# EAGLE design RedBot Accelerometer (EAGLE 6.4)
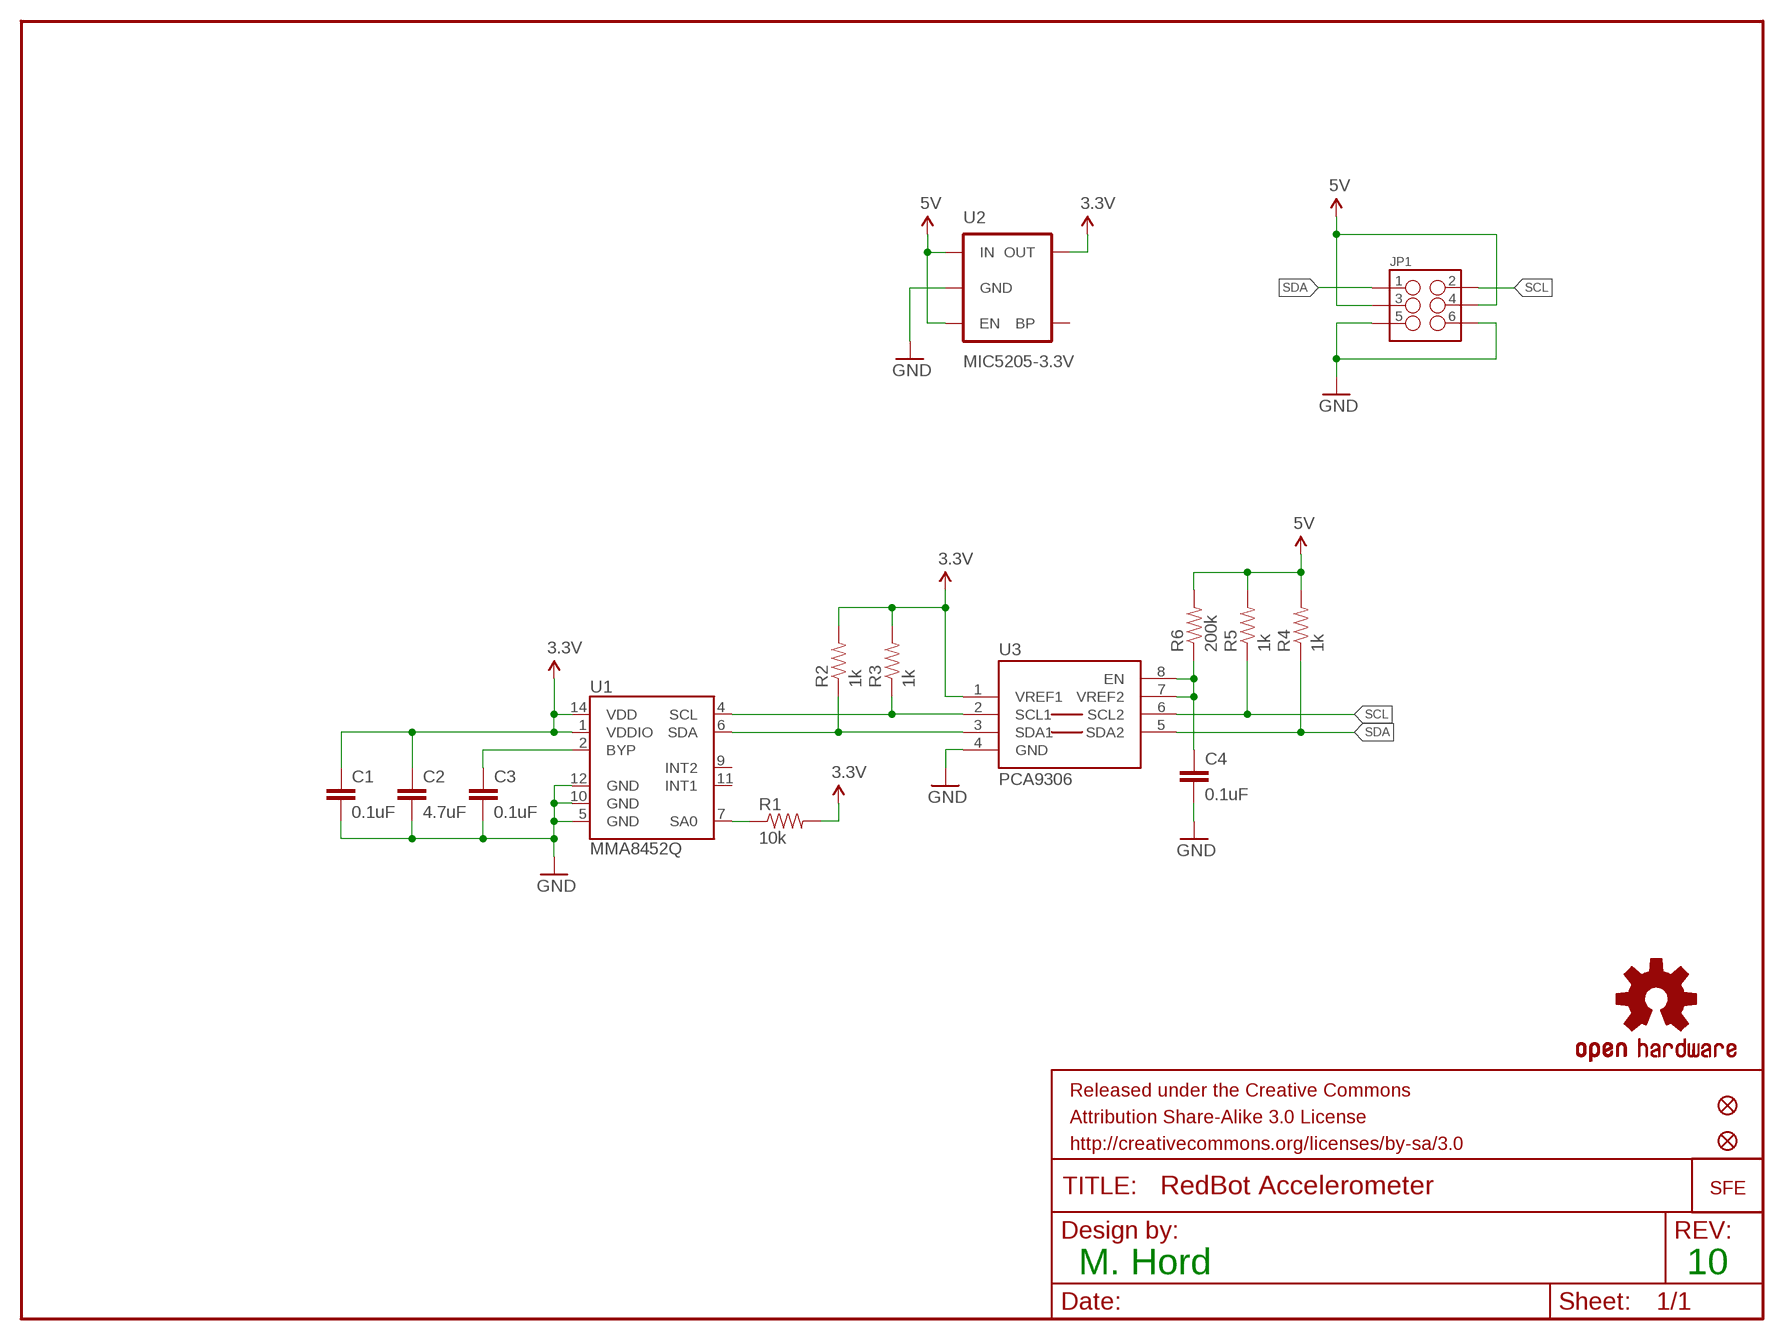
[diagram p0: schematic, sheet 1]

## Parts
C1  0.1uF  0.1UF-25V(+80/-20%)(0603)  [0402-CAP]
C2  4.7uF  4.7UF-6.3V-10%(0603)  [0402-CAP]
C3  0.1uF  0.1UF-25V(+80/-20%)(0603)  [0402-CAP]
C4  0.1uF  0.1UF-25V(+80/-20%)(0603)  [0402-CAP]
FID1  FIDUCIALUFIDUCIAL  [MICRO-FIDUCIAL]
FID2  FIDUCIALUFIDUCIAL  [MICRO-FIDUCIAL]
FRAME1  FRAME-LETTER  [CREATIVE_COMMONS]
JP1  M03X2NO_SILK  [2X3-NS]
LOGO1  LOGO-SFESK  [SFE-LOGO-FLAME]
LOGO2  OSHW-LOGOS  [OSHW-LOGO-S]
R1  10k  10KOHM1/10W1%(0603)  [0402-RES]
R2  1k  1K-1%  [0402-RES]
R3  1k  1K-1%  [0402-RES]
R4  1k  1K-1%  [0402-RES]
R5  1k  1K-1%  [0402-RES]
R6  200k  200KOHM1/10W1%(0603)200K  [0402-RES]
U1  MMA8452Q  [QFN-16_0.5MM]
U2  MIC5205-3.3V  MIC52053.3V  [SOT23-5]
U3  PCA9306  [PSOP-8]

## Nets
3.3V: C1.1 C2.1 R1.2 R2.2 R3.2 U1.1(VDDIO) U1.14(VDD) U2.5(OUT) U3.1(VREF1)
5V: JP1.3 JP1.4 R4.2 R5.2 R6.2 U2.1(IN) U2.3(EN)
ADDR: R1.1 U1.7(SA0)
GND: C1.2 C2.2 C3.2 C4.2 JP1.5 JP1.6 U1.5(GND) U1.10(GND) U1.12(GND) U2.2(GND) U3.4(GND)
N$1: C3.1 U1.2(BYP)
N$2: C4.1 R6.1 U3.7(VREF2) U3.8(EN)
SCL: JP1.2 R5.1 U3.6(SCL2)
SCL1: R3.1 U1.4(SCL) U3.2(SCL1)
SDA: JP1.1 R4.1 U3.5(SDA2)
SDA1: R2.1 U1.6(SDA) U3.3(SDA1)
Unconnected: U1.9(INT2) U1.11(INT1) U2.4(BP)

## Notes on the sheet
- M. Hord | 10

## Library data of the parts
C1 C3 C4 = SparkFun-Capacitors:0.1UF-25V(+80/-20%)(0603): Ceramic; PROD_ID: CAP-00810
C2 = SparkFun-Capacitors:4.7UF-6.3V-10%(0603): CAP-08280; PROD_ID: CAP-08280
FID1 FID2 = SparkFun-Aesthetics:FIDUCIAL: Fiducial Alignment Points
FRAME1 = SparkFun-Aesthetics:FRAME-LETTER: Schematic Frame
JP1 = SparkFun-Connectors:M03X2: 2x3 .1" header. Shrouded, with keying- CONN-10681 SMT- CONN-11415 Pogo pins- HW-11044
LOGO1 = SparkFun-Aesthetics:LOGO-SFE: Spark Fun Electronics PCB Logo
LOGO2 = SparkFun-Aesthetics:OSHW-LOGO: Open Source Hardware Logo This logo indicates the piece of hardware it is found on incorporates a OSHW license and/or adheres to the definition of open source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
R1 = SparkFun-Resistors:10KOHM1/10W1%(0603): RES-00824; PROD_ID: RES-00824
R2-R5 = SparkFun-Resistors:1K-1%: 1k-ohm SMT; PROD_ID: RES-07856
R6 = SparkFun-Resistors:200KOHM1/10W1%(0603): RES-09385; PROD_ID: RES-09385
U1 = SparkFun-Sensors:MMA8452Q: MMA8452Q 3-Axis, 12/8-bit Digital Accelerometer Supply Voltage: 1.6-3.6V Range: +/- 2g, 4g, 8g Interface: I2C, 12-bit and 8-bit ODR: 1.56 Hz - 800 Hz Package: QFN-16 http://cache.freescale.com/files/sensors/doc/data_sheet/MMA8452Q.pdf; PROD_ID: IC-10769
U2 = SparkFun-PowerIC:MIC5205: MIC5205 150mA vreg 3.3V - VREG-00822 5V - VREG-00823; PROD_ID: VREG-00822
U3 = SparkFun-DigitalIC:PCA9306: Bidirectional I2C level shifter. NOT compatible with all available part number pinout schemes- DOUBLE CHECK!!!; PROD_ID: IC-10023

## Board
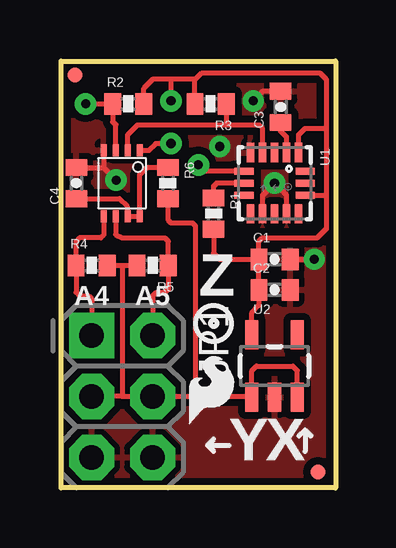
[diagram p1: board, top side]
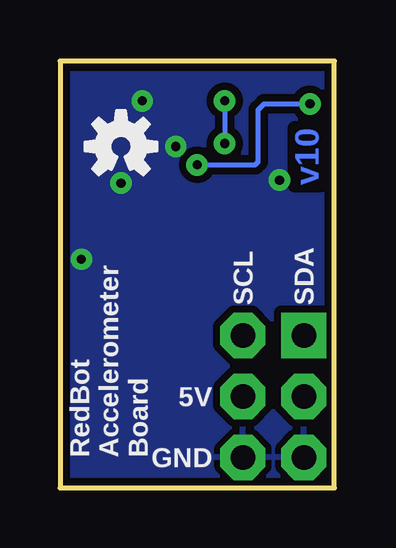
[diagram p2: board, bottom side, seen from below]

Size 11.43 x 17.78 mm. Coordinates in mm from the lower left corner, seen from the top.
Outline: 0,0 0,17.78 11.43,17.78 11.43,0 0,0
Copper layers (1*16): Top 0.035mm / dielectric 1.5mm / Bottom 0.035mm
Design rules "Sparkfun": minimum track width 8mil, minimum drill 20mil, track to track 8mil, track to pad 8mil, pad to pad 8mil, via to via 8mil, smd to smd 8mil, copper to edge 8mil, drill to drill 8mil, minimum pad ring 12mil, minimum via ring 10mil, stop-mask expansion 4mil, vias tented up to drill 20mil, thermal gap 10mil

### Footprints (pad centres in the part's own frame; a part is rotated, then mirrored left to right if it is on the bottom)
0402-CAP = smd 0.7 x 0.9: 1 -0.65,0; 2 0.65,0
MICRO-FIDUCIAL = smd 0.635 x 0.635: 1 0,0
2X3-NS = drill 1.016 pad 1.88 square: 1 -2.54,-1.27 | drill 1.016 pad 1.88 octagon: 2 -2.54,1.27; 3 0,-1.27; 4 0,1.27; 5 2.54,-1.27; 6 2.54,1.27
0402-RES = smd 0.7 x 0.9: 1 -0.65,0; 2 0.65,0
QFN-16_0.5MM = smd 0.8 x 0.3: 1 -1.275,1; 2 -1.275,0.5; 3 -1.275,0; 4 -1.275,-0.5; 5 -1.275,-1; 9 1.275,-1; 10 1.275,-0.5; 11 1.275,0; 12 1.275,0.5; 13 1.275,1 | smd 0.3 x 0.8: 6 -0.5,-1.275; 7 0,-1.275; 8 0.5,-1.275; 14 0.5,1.275; 15 0,1.275; 16 -0.5,1.275
SOT23-5 = smd 0.55 x 1.2: 1 -0.95,-1.3; 2 0,-1.3; 3 0.95,-1.3; 4 0.95,1.3; 5 -0.95,1.3
PSOP-8 = smd 0.25 x 0.5: 1 -0.73,-1.37; 2 -0.23,-1.37; 3 0.27,-1.37; 4 0.77,-1.37; 5 0.77,1.38; 6 0.27,1.38; 7 -0.23,1.38; 8 -0.73,1.38

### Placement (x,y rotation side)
C1  8.89,9.53 0 top
C2  8.89,8.26 0 top
C3  9.14,15.88 90 top
C4  0.64,12.7 90 top
FID1  0.58,17.2 0 top
FID2  10.69,0.66 0 top
FRAME1  not placed on the board
JP1  2.54,3.81 270 top
LOGO1  5.33,2.67 0 top
LOGO2  8.89,14.22 0 bottom
R1  6.35,11.43 270 top
R2  2.79,16 0 top
R3  6.22,16 180 top
R4  1.27,9.27 0 top
R5  3.81,9.27 180 top
R6  4.45,12.7 270 top
U1  8.89,12.7 270 top
U2  8.89,5.08 0 top
U3  2.54,12.7 180 top

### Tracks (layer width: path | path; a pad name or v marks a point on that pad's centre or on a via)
3.3V  (via drill 0.38)
  Top 0.203: U2.5 7.94,7.3 8.24,7.61 C2.1 C1.1 | R1.2 6.35,9.78 6.6,9.53 C1.1 | C1.1 8.24,10.27 8.38,10.41 10.67,10.41 11.05,10.79 11.05,12.19 | U1.14 11.04,12.2 11.05,12.19 | U1.1 9.89,14.72 10.16,14.99 11.05,14.99 | 11.05,14.99 11.05,17.02 10.79,17.27 5.84,17.27 5.59,17.02 | 11.05,14.99 11.05,12.19 | 5.59,17.02 4.57,17.02 | 4.57,17.02 3.81,17.02 3.44,16.65 R2.2 | R3.2 5.57,17 5.59,17.02 | 4.57,17.02 v4.57,16.13 | v4.57,14.35 3.94,14.35 3.66,14.07 U3.1
  Bottom 0.203: v4.57,16.13 v4.57,14.35
5V
  Top 0.203: R4.2 2.54,9.27 | 2.54,9.27 R5.2 | 2.54,9.27 2.54,3.81 | 2.54,3.81 JP1.3 | 2.54,3.81 JP1.4 5.59,3.81 | R6.2 4.45,11.18 4.57,11.05 5.46,11.05 5.59,10.92 5.59,3.81 | U2.3 9.84,4.89 9.65,5.08 8.13,5.08 7.94,4.89 U2.1 7.91,3.81 5.59,3.81
ADDR
  Top 0.203: R1.1 6.35,12.57 6.48,12.7 U1.7
GND  (via drill 0.38)
  Top 0.203: U3.4 1.77,13.34 v2.29,12.83 1.76,13.35 C4.2 | C1.2 v10.54,9.53 | U1.12 9.39,12.2 v8.89,12.7 8.39,12.2 U1.10 | C3.2 8.4,16.52 v8,16.13
  other vias: 6.6,14.22
  pour Top (isolate 0.305): 0,17.78 11.43,17.78 11.43,0 0,0
  pour Bottom (isolate 0.305): 0,17.78 11.43,17.78 11.43,0 0,0
N$1
  Top 0.203: U1.2 9.39,14.61 9.14,14.86 C3.1
N$2
  Top 0.203: C4.1 2.43,12.05 2.77,11.71 U3.7 U3.8 3.27,13.05 3.57,13.35 R6.1
SCL
  Top 0.203: U3.6 2.27,10.56 2.54,10.41 4.32,10.41 4.46,10.27 R5.1 4.46,8.27 4.32,8.13 3.94,8.13 3.81,8 JP1.2
SCL1
  Top 0.203: U1.4 8.39,14.98 8.26,15.11 6.86,15.11 | 6.86,15.11 5.33,15.11 | 5.33,15.11 3.17,15.11 2.77,14.71 U3.2 | 5.32,15.13 5.33,15.11 | R3.1 6.87,15.13 6.86,15.11
SDA
  Top 0.203: U3.5 1.77,10.53 1.65,10.41 0.76,10.41 0.62,10.27 R4.1 0.62,8.14 0.76,8 1.14,8 1.27,7.87 JP1.1
SDA1  (via drill 0.38)
  Top 0.203: U3.3 2.27,15.1 2.29,15.11 2.14,15.26 R2.1 v1.02,16 | U1.6 5.98,13.2 v5.71,13.46
  Bottom 0.203: v5.71,13.46 3.3,13.46 3.17,13.59 3.17,15.75 2.92,16 v1.02,16

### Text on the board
Bottom: v10
tPlace: A4 | A5 | Z | Y | X
bPlace: SDA | SCL | 5V | GND | RedBot / Accelerometer / Board
tValues: M. Hord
